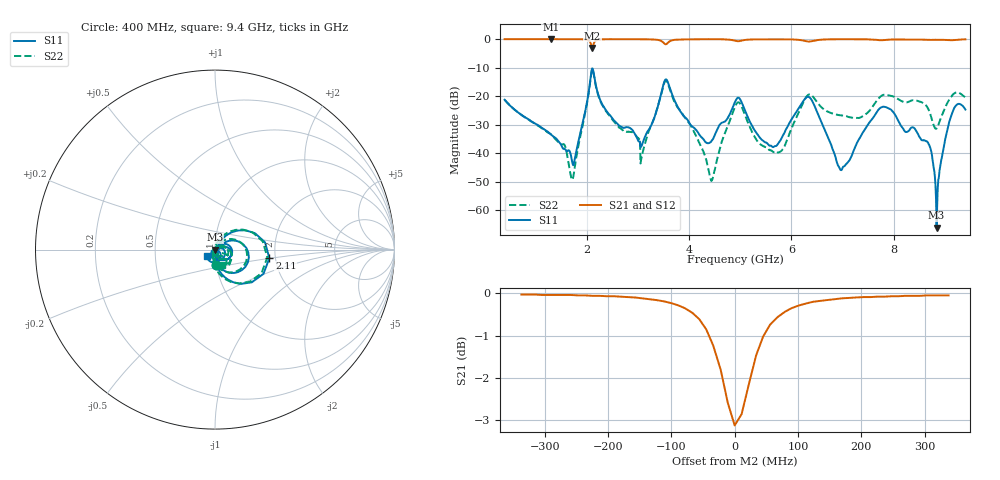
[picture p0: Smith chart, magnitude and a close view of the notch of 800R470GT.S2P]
!  American Technical Ceramics  Date:  6/19/09
!  One Norden Lane
!  Huntington Station,  NY.  11746-2102
!  Tel:  (631) 622-4700  Fax:  (631) 622-4748
!  Part Number  800R470GT
!  Description: Ultra-low ESR, NPO  Mounting Orientation: Horizontal
!  Application: High RF power Filters, Combiners, Matching networks,
!  Antenna, DC block, Bypass and Couplers
# GHZ S DB R 50
! Freq  |S11|  S11 Ph  |S21|  S21 Ph  |S12|  S12 Ph  |S22|  S22 Ph
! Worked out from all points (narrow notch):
!   801 points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, 400 MHz to 9.4 GHz, reference 50 ohm
!   highest |S21| = -0.01 dB at 1.3 GHz (marker M1); lowest = -3.1 dB at 2.11 GHz (marker M2)
!   notch at M2: 3.0 dB deep, 57.4 MHz wide at half that depth
!   lowest |S11| = -66.2 dB at 8.838 GHz (marker M3), VSWR 1.00, Z = 50 - j0.044 ohm
!   |S11| at or under -10 dB: start of sweep to end of sweep
!   |S22| runs from -49.8 to -10.6 dB; largest |S21 - S12| = 0.0051
!   S11 on the Smith chart (normalised r, x): 400 MHz: 1.00, -0.17; 2.11 GHz: 1.86, -0.19; 9.4 GHz: 0.91, -0.07
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0.4  -21.29 -86.2  -0.03 3.0  -0.06 3.0  -21.29 -86.6
1.3  -33.36 -84.2  -0.01 -5.0  -0.04 -5.0  -33.36 -99.9
1.57  -38.56 -59.2  -0.03 -6.8  -0.05 -6.8  -37.14 -111.4
1.716  -42.79 -35.4  -0.04 -8.0  -0.06 -8.0  -49.37 161.2
1.908  -30.80 54.0  -0.07 -10.4  -0.09 -10.3  -31.69 77.5
2.11  -10.27 -8.8  -3.12 -10.4  -3.15 -10.3  -10.61 -8.4
2.391  -25.28 -85.0  -0.06 -8.0  -0.08 -8.0  -25.57 -103.0
3.1  -36.23 2.3  -0.06 -13.9  -0.08 -13.8  -39.55 79.3
3.404  -22.97 35.5  -0.33 -18.2  -0.35 -18.1  -23.00 46.4
3.573  -14.51 -37.5  -1.59 -10.6  -1.61 -10.5  -15.00 -38.5
3.876  -26.54 -79.1  -0.14 -13.8  -0.16 -13.7  -26.35 -102.5
4.439  -35.86 -4.7  -0.05 -18.2  -0.07 -18.1  -49.79 158.6
4.9  -22.05 4.0  -0.57 -22.1  -0.58 -22.0  -23.78 8.8
5.733  -36.92 23.8  -0.10 -23.6  -0.10 -23.4  -39.80 -24.6
6.408  -21.71 -44.7  -0.71 -23.8  -0.71 -23.6  -19.90 -54.6
6.97  -46.00 -25.1  -0.06 -27.6  -0.05 -27.4  -26.77 -74.9
7.701  -24.82 -13.4  -0.35 -32.2  -0.34 -32.0  -20.93 -44.9
7.904  -24.35 -76.2  -0.20 -31.2  -0.19 -31.0  -19.75 -71.0
8.669  -36.30 -158.0  -0.28 -35.2  -0.26 -35.0  -24.31 -101.4
8.838  -66.19 -116.0  -0.25 -35.3  -0.23 -35.1  -31.37 -58.1
9.13  -26.58 -46.4  -0.41 -35.4  -0.39 -35.2  -20.03 -31.6
9.4  -24.74 -138.7  -0.09 -35.1  -0.07 -34.9  -20.52 -63.9
